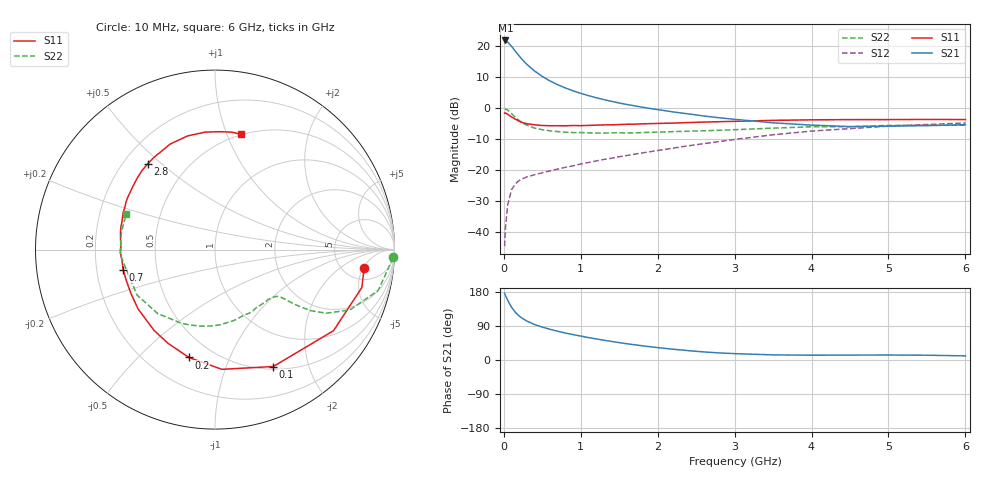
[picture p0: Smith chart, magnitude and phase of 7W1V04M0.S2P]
! Infineon Technologies  Discrete & RF Semiconductors
! BFS17W
! Si NPN RF Bipolar Junction Transistor in SOT323
! VCE = 1 V  IC = 4 mA
! Common Emitter S-Parameters:  August  1999
# GHz  S  MA  R  50
!  f  S11  S21  S12  S22
! GHz  MAG  ANG  MAG  ANG  MAG  ANG  MAG  ANG
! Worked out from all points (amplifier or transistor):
!   36 points, 10 MHz to 6 GHz, reference 50 ohm
!   highest |S21| = 22.0 dB at 20 MHz (marker M1)
!   |S21| within 3 dB of that: start of sweep to 134.5 MHz
!   unconditionally stable (mu >= 1): 557.1 MHz to end of sweep
!   at 250 MHz: K = 0.55, MSG = 19.1 dB, |S12| = -22.7 dB
!   at 1.4 GHz: K = 1.36, MAG = 5.6 dB, |S12| = -16.1 dB
!   at 6 GHz: K = 1.12, MAG = -2.4 dB, |S12| = -4.7 dB
!   S11 on the Smith chart (normalised r, x): 10 MHz: 7.67, -5.23; 100 MHz: 0.53, -1.48; 200 MHz: 0.37, -0.72; 700 MHz: 0.32, -0.10; 2.8 GHz: 0.30, +0.45; 6 GHz: 0.50, +1.13
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0.01  0.8371 -7.0  12.49 176.0  0.0059 84.6  0.9914 -2.5
0.02  0.845 -14.5  12.52 170.7  0.0114 80.9  0.9729 -5.9
0.05  0.8001 -34.4  11.76 157.3  0.0275 72.0  0.9369 -14.1
0.1  0.7278 -63.5  10.05 139.3  0.0483 60.0  0.8231 -24.1
0.15  0.6682 -86.7  8.372 125.6  0.06 50.5  0.7134 -29.8
0.2  0.6184 -103.6  7.012 115.9  0.0681 46.1  0.6333 -32.5
0.25  0.5838 -116.7  5.938 108.6  0.0733 42.6  0.5727 -33.8
0.3  0.564 -127.0  5.132 102.8  0.0777 42.0  0.533 -34.6
0.4  0.5411 -142.5  4.011 93.6  0.0845 41.2  0.4785 -35.3
0.5  0.5278 -153.1  3.279 86.8  0.0906 42.4  0.4514 -35.9
0.6  0.5232 -161.3  2.77 81.0  0.0973 43.9  0.4326 -37.0
0.7  0.5238 -167.7  2.411 75.9  0.1041 45.5  0.4207 -38.9
0.9  0.5267 -178.1  1.918 67.1  0.1175 48.1  0.4059 -43.3
1.1  0.5297 173.5  1.604 59.1  0.1332 50.2  0.4013 -48.9
1.3  0.5398 166.3  1.384 52.2  0.1492 51.7  0.3976 -55.3
1.6  0.5524 157.6  1.153 42.9  0.1726 53.5  0.3996 -65.2
2.2  0.5774 142.3  0.875 28.4  0.2272 55.1  0.4198 -86.2
2.8  0.6078 128.0  0.704 18.7  0.2903 53.7  0.4416 -107.7
3.5  0.639 112.9  0.583 13.5  0.3737 48.8  0.4784 -131.8
4.5  0.6569 94.8  0.507 13.0  0.4695 37.4  0.503 -164.9
5.5  0.6611 81.9  0.525 12.6  0.5473 26.5  0.5308 169.4
6  0.6586 77.1  0.544 10.9  0.5791 21.2  0.5327 158.1
